FUNCTION_BLOCK EventController
VAR_IN_OUT
	eventData: ST_event;
END_VAR
VAR_INPUT
	raise: bool;
	confirm: bool;
	clear: bool;
	reset: bool;
END_VAR
VAR
	fbTime: FB_LocalSystemTime := (bEnable := TRUE, dwCycle := 1);
	currTime: TIMESTRUCT;
END_VAR

// FB for state control of an event
// States:
// 0 - INACTIVE
// 1 - RAISED
// 2 - CONFIRMED

// Get current time
fbTime();

IF reset THEN	
	eventData.state := 0;
	eventData.timestamp_raised := DT#1970-1-1-0:0;
	eventData.timestamp_confirmed := DT#1970-1-1-0:0;
	
ELSE
	
	CASE eventData.state OF
		0:  // INACTIVE
			IF raise THEN
				
				currTime := fbTime.systemTime;
				eventData.timestamp_raised := SYSTEMTIME_TO_DT(TIMESTR := currTime);
				IF eventData.needs_confirmation THEN
					eventData.state := 1;
				ELSE
					eventData.state := 3;
				END_IF
			END_IF
		1:  // RAISED (confirmable)
			// If confirmation is needed and we get the confirm signal, we change state to CONFIRMED
			IF confirm THEN
				eventData.state := 2;
				eventData.timestamp_confirmed := SYSTEMTIME_TO_DT(TIMESTR := currTime);
			END_IF
		2:  // CONFIRMED (confirmable)
			// Change state to INACTIVE if clear signal is high and raise is low
			IF clear AND NOT raise THEN
				eventData.state := 0;
			END_IF
		3:  // ACTIVE (non-confirmable)
			// If confirmation is not required, we can clear the event on a high clear input and transit to INACTIVE state
			IF clear AND NOT raise THEN
				eventData.state := 0;
			END_IF
		
		ELSE
			eventData.state := 0;
		
	END_CASE
END_IF

END_FUNCTION_BLOCK
